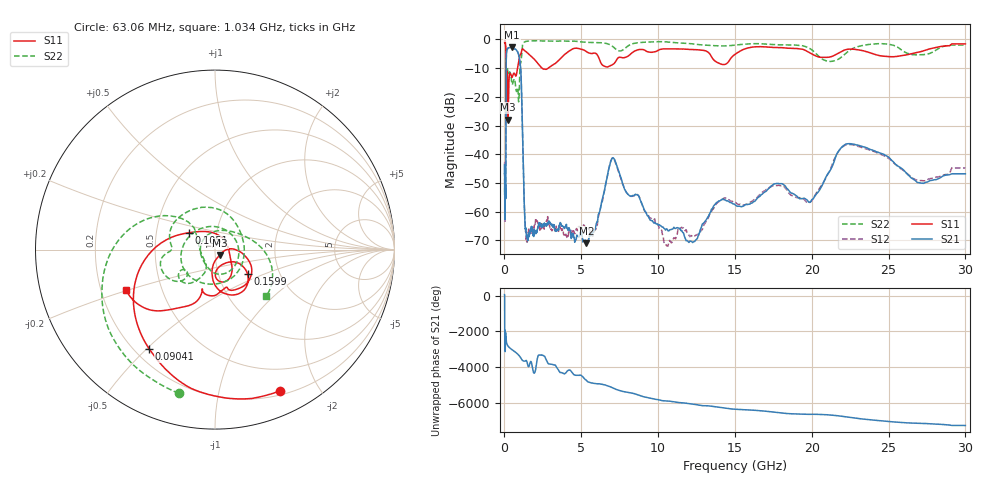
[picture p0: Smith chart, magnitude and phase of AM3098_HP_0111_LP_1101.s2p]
! Date/Time: Thu, Feb 28, 2019 8:39 AM
! Network Analyzer: Agilent Technologies E8364B Rev: A.07.50.67
! Sweep from 0.010 to 30.000 GHz, 1601 Points, Sweep Type: LOG
! Power Supply: 5.022 V, 0.002 A
# Hz S DB R 50
!freq MagS11 AngS11 MagS21 AngS21 MagS12 AngS12 MagS22 AngS22
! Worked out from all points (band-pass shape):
!   1601 points, 10 MHz to 30 GHz, reference 50 ohm
!   highest |S21| = -2.80 dB at 490.6 MHz (marker M1); lowest = -71.0 dB at 5.338 GHz (marker M2)
!   |S21| within 3 dB of the highest: 122.2 MHz to 945.1 MHz (822.8 MHz wide, 154 % of centre)
!   lowest |S11| = -27.9 dB at 237.5 MHz (marker M3), VSWR 1.08, Z = 52.7 - j3.1 ohm
!   |S11| at or under -10 dB: 102.2 MHz to 849.5 MHz (747.3 MHz wide, 157 % of centre); 2.452 GHz to 2.844 GHz (391.8 MHz wide, 14.8 % of centre)
!   |S22| runs from -22.1 to -0.4 dB; largest |S21 - S12| = 0.011
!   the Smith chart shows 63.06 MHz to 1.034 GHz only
!   S11 on the Smith chart (normalised r, x): 63.06 MHz: 0.24, -1.53; 90.41 MHz: 0.26, -0.51; 105.1 MHz: 0.74, +0.14; 159.9 MHz: 1.38, -0.40; 1.034 GHz: 0.31, -0.20
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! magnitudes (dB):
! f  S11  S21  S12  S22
! 10 MHz  -0.3  -46.9  -42.9  -0.6
! 38.04 MHz  -0.5  -60.7  -61.9  -1.0
! 63.06 MHz  -1.2  -52.8  -53.3  -1.7
! 90.41 MHz  -3.6  -46.4  -45.0  -3.9
! 105.1 MHz  -15.3  -14.9  -14.9  -19.8
! 144.7 MHz  -19.8  -4.0  -4.0  -14.0
! 159.9 MHz  -12.9  -3.7  -3.6  -11.7
! 237.5 MHz  -27.9  -3.0  -2.9  -12.1
! 311.2 MHz  -12.9  -2.9  -2.8  -11.5
! 490.6 MHz  -13.2  -2.8  -2.8  -15.6
! 550.5 MHz  -12.5  -3.0  -3.0  -15.0
! 926.3 MHz  -7.8  -5.4  -5.3  -21.7
! 1.034 GHz  -5.3  -8.9  -8.8  -8.3
! 1.396 GHz  -4.2  -66.1  -67.6  -0.7
! 2.084 GHz  -7.7  -67.0  -63.0  -0.5
! 5.338 GHz  -4.3  -71.0  -66.0  -1.0
! 6.994 GHz  -8.9  -41.5  -41.5  -2.2
! 7.926 GHz  -6.1  -53.2  -53.3  -2.7
! 10.76 GHz  -3.3  -66.3  -70.0  -1.0
! 19.8 GHz  -4.5  -56.7  -56.9  -3.0
! 22.67 GHz  -3.4  -36.5  -36.7  -3.2
! 30 GHz  -1.5  -46.8  -44.8  -1.9
